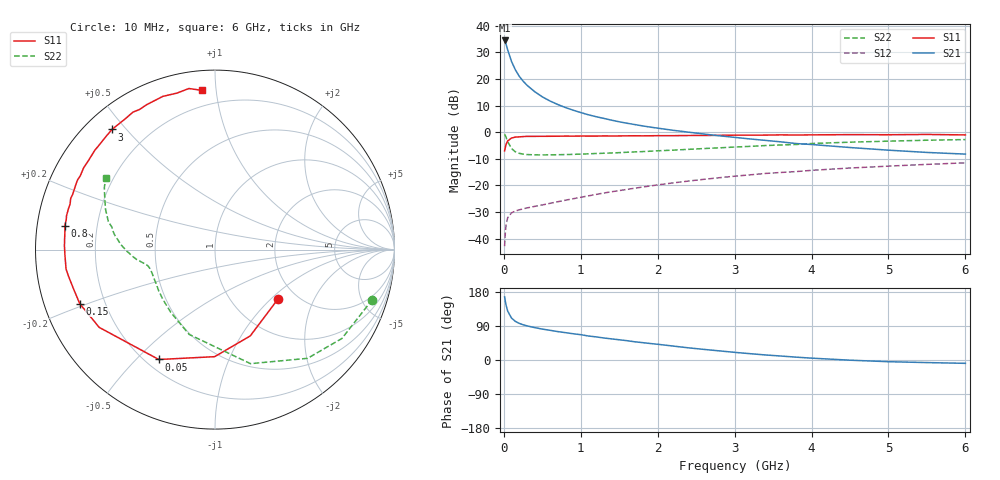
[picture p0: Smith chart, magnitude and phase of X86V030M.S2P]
! SIEMENS Small Signal Semiconductors
! BFP136W
! Si NPN RF Bipolar Junction Transistor in SOT343
! VCE = 6 V  IC = 30 mA
! Common Emitter S-Parameters:  September  1994
# GHz  S  MA  R  50
!  f  S11  S21  S12  S22
! GHz  MAG  ANG  MAG  ANG  MAG  ANG  MAG  ANG
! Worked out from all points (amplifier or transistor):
!   40 points, 10 MHz to 6 GHz, reference 50 ohm
!   highest |S21| = 34.5 dB at 10 MHz (marker M1)
!   |S21| within 3 dB of that: start of sweep to 44.65 MHz
!   unconditionally stable (mu >= 1): 853.5 MHz to 2.836 GHz
!   at 200 MHz: K = 0.42, MSG = 25.1 dB, |S12| = -29.2 dB
!   at 1.5 GHz: K = 1.13, MAG = 10.8 dB, |S12| = -21.9 dB
!   at 6 GHz: K = 0.96, MSG = 1.6 dB, |S12| = -11.5 dB
!   S11 on the Smith chart (normalised r, x): 10 MHz: 1.61, -1.11; 50 MHz: 0.25, -0.58; 150 MHz: 0.11, -0.19; 800 MHz: 0.08, +0.08; 3 GHz: 0.08, +0.46; 6 GHz: 0.11, +0.91
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0.01  0.4461 -38.2  53.25 166.6  0.0072 76.2  0.9199 -17.6
0.02  0.5196 -67.8  49.09 154.1  0.0133 66.5  0.8633 -35.0
0.03  0.5966 -90.2  44.82 144.1  0.0184 57.7  0.7955 -49.6
0.05  0.6878 -117.1  35.39 129.0  0.0247 44.1  0.6656 -72.7
0.1  0.7771 -146.1  21.41 110.6  0.0305 32.4  0.4942 -106.9
0.15  0.8116 -158.2  14.92 101.9  0.033 29.3  0.428 -125.1
0.2  0.8185 -164.8  11.32 96.7  0.0347 28.6  0.4013 -136.4
0.25  0.829 -169.5  9.174 93.0  0.0362 29.6  0.3889 -143.6
0.3  0.8368 -172.5  7.689 90.2  0.0377 30.3  0.3806 -148.7
0.4  0.8366 -177.6  5.808 85.5  0.0403 32.7  0.3756 -155.3
0.5  0.839 178.7  4.636 81.6  0.0429 35.4  0.3745 -159.5
0.6  0.84 175.9  3.866 78.4  0.046 38.2  0.3757 -162.0
0.7  0.8422 173.0  3.329 75.0  0.0493 41.1  0.3779 -163.7
0.8  0.847 171.0  2.916 72.2  0.0527 43.0  0.3805 -165.0
1.1  0.8476 164.2  2.128 63.3  0.0636 47.7  0.3927 -167.7
1.6  0.8558 155.0  1.478 51.0  0.0841 51.5  0.4201 -170.9
2.2  0.8622 144.5  1.088 36.8  0.1114 51.5  0.4607 -175.3
3  0.8816 130.6  0.801 20.2  0.1491 47.4  0.5266 176.8
3.2  0.8816 127.1  0.748 16.7  0.158 45.9  0.5427 174.4
4.5  0.9018 108.8  0.516 -0.5  0.2123 35.4  0.6505 159.7
5.5  0.9091 99.2  0.417 -6.8  0.2486 27.3  0.7082 150.5
6  0.8905 94.8  0.388 -8.8  0.266 22.8  0.728 146.6
